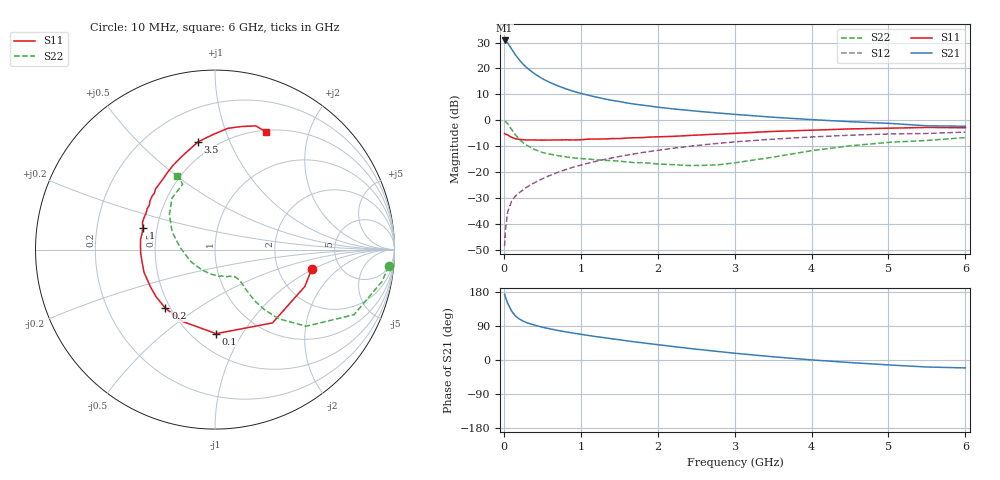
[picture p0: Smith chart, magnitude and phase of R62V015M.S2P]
! SIEMENS Small Signal Semiconductors
! BFR193
! Si NPN RF Bipolar Junction Transistor in SOT23
! VCE = 2 V  IC = 15 mA
! Common Emitter S-Parameters:  May  1996
# GHz  S  MA  R  50
!  f  S11  S21  S12  S22
! GHz  MAG  ANG  MAG  ANG  MAG  ANG  MAG  ANG
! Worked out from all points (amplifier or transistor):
!   36 points, 10 MHz to 6 GHz, reference 50 ohm
!   highest |S21| = 30.8 dB at 10 MHz (marker M1)
!   |S21| within 3 dB of that: start of sweep to 94 MHz
!   unconditionally stable (mu >= 1): 606.6 MHz to 1.894 GHz; 1.943 GHz to 2.015 GHz
!   at 250 MHz: K = 0.77, MSG = 24.2 dB, |S12| = -26.9 dB
!   at 1.4 GHz: K = 1.03, MAG = 10.1 dB, |S12| = -14.6 dB
!   at 6 GHz: K = 0.95, MSG = 1.1 dB, |S12| = -4.6 dB
!   S11 on the Smith chart (normalised r, x): 10 MHz: 3.11, -0.96; 100 MHz: 0.65, -0.78; 200 MHz: 0.47, -0.38; 1 GHz: 0.42, +0.12; 3.5 GHz: 0.40, +0.77; 6 GHz: 0.52, +1.40
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0.01  0.5498 -11.3  34.67 173.4  0.0037 84.4  0.9715 -5.5
0.02  0.541 -22.3  34.34 166.7  0.0075 79.4  0.9473 -10.8
0.05  0.5191 -51.9  31.05 149.6  0.017 71.3  0.8553 -25.1
0.1  0.4684 -89.3  23.77 129.4  0.0272 62.2  0.6631 -40.1
0.15  0.439 -114.3  18.3 116.4  0.0343 59.1  0.5232 -47.4
0.2  0.428 -130.2  14.65 108.4  0.0398 59.2  0.4303 -50.6
0.25  0.4205 -141.2  12.05 102.7  0.0453 59.8  0.3685 -52.0
0.3  0.4152 -149.8  10.24 98.2  0.0512 61.3  0.3274 -52.3
0.4  0.4153 -162.2  7.886 92.0  0.0622 63.8  0.2717 -52.1
0.5  0.4122 -170.3  6.343 86.6  0.0739 65.1  0.2391 -51.5
0.6  0.4146 -177.4  5.343 82.2  0.086 65.5  0.2211 -51.4
0.7  0.4156 177.3  4.634 78.1  0.0983 66.1  0.2075 -52.0
0.8  0.4188 172.2  4.064 74.4  0.111 65.9  0.1965 -52.8
1  0.4195 163.4  3.299 67.9  0.1358 65.3  0.1822 -55.2
1.1  0.4312 159.6  3.031 64.7  0.1487 64.7  0.1777 -57.8
1.4  0.4414 148.9  2.425 56.1  0.1865 62.1  0.1662 -65.1
1.6  0.453 143.1  2.155 50.6  0.212 59.8  0.1566 -72.2
2.2  0.4882 126.5  1.655 35.6  0.2874 52.4  0.1387 -99.5
3.5  0.6077 98.9  1.142 8.5  0.4313 32.9  0.1935 177.0
4.5  0.6792 84.0  0.937 -6.7  0.5143 18.4  0.3206 142.4
5.5  0.7257 71.8  0.78 -18.5  0.5543 3.7  0.4068 116.3
6  0.7151 66.4  0.765 -20.9  0.5909 -0.6  0.4618 116.9
